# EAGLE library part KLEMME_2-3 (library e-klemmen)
Klemme 2 3
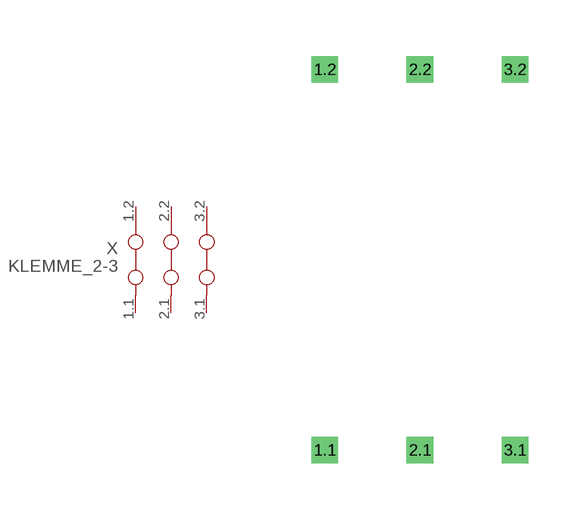
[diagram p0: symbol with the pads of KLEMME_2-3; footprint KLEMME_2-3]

Designator prefix X

## KLEMME_2-3  [KLEMME_2-3]
1.1  1.1  pas
1.2  1.2  pas
2.1  2.1  pas
2.2  2.2  pas
3.1  3.1  pas
3.2  3.2  pas

## Footprint KLEMME_2-3 (pad centres in mm)
Dummy
drill 0.2 pad 0.6 square: 1.1 -2.54,-5.08; 1.2 -2.54,5.08; 2.1 0,-5.08; 2.2 0,5.08; 3.1 2.54,-5.08; 3.2 2.54,5.08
